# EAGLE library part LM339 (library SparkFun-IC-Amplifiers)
Quad Comparator - LM339PWR Based on information from the SLCS006N datasheet from TI (www.ti.com). Created by nick@scantool.net, 2008. Updated 2016. SparkFun Products SparkFun OBD-II UART (WIG-09555) SparkFun Car Diagnostics Kit (RTL-10769)
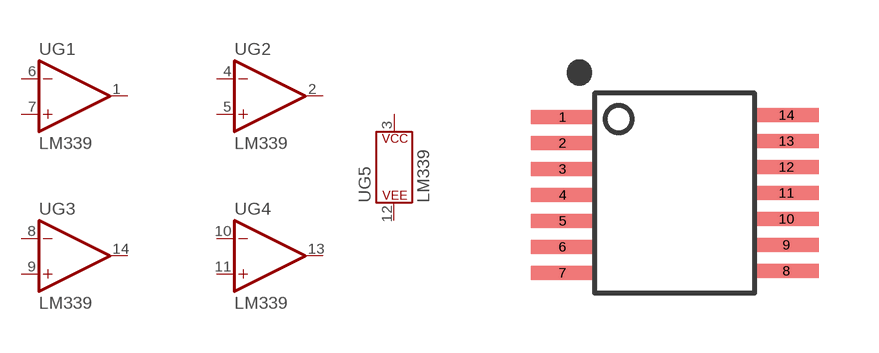
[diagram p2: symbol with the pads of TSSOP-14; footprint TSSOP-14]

Designator prefix U; gates G1=OP-AMP G2=OP-AMP G3=OP-AMP G4=OP-AMP G5=POWER_CONSORT

## LM339 (PROD_ID: IC-09990; VALUE: LM339PWR)  [TSSOP-14]
1  G1:OUT  out
2  G2:OUT  out
3  G5:P$V+
4  G2:-IN  in
5  G2:+IN  in
6  G1:-IN  in
7  G1:+IN  in
8  G3:-IN  in
9  G3:+IN  in
10  G4:-IN  in
11  G4:+IN  in
12  G5:P$V-
13  G4:OUT  out
14  G3:OUT  out

## Footprint TSSOP-14 (pad centres in mm)
smd 1.6 x 0.35: 1 -2.8,1.9; 2 -2.8,1.25; 3 -2.8,0.6; 4 -2.8,-0.05; 5 -2.8,-0.7; 6 -2.8,-1.35; 7 -2.8,-2; 8 2.8,-1.95; 9 2.8,-1.3; 10 2.8,-0.65; 11 2.8,0; 12 2.8,0.65; 13 2.8,1.3; 14 2.8,1.95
